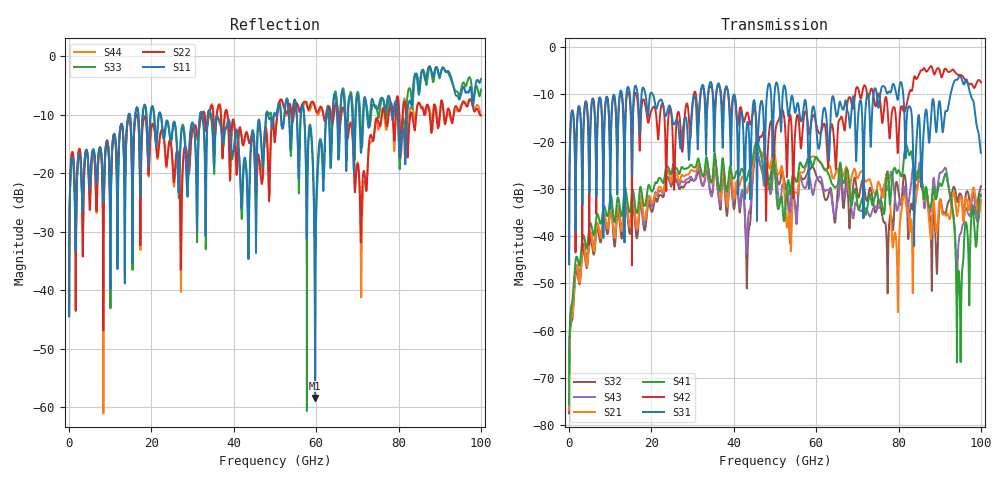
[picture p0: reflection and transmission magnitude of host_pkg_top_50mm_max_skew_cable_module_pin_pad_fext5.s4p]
# Hz S RI R 50
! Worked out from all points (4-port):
!   10000 points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, 10 MHz to 100 GHz, reference 50 ohm
!   strongest paths, dB at 10 MHz, 25.01 GHz, 50.01 GHz, 75.01 GHz, 100 GHz:
!     S31: -46.0, -15.0, -8.7, -12.4, -22.4
!     S42: -45.9, -16.0, -18.9, -10.1, -7.5
!     S41: -75.7, -26.1, -26.6, -32.0, -31.5
!     S21: -76.7, -27.8, -23.0, -28.6, -32.6
!     S43: -76.8, -28.1, -25.4, -34.0, -32.4
!     S32: -77.5, -28.8, -24.1, -32.7, -29.5
!   lowest |S11| = -58.4 dB at 59.73 GHz (marker M1), VSWR 1.00, Z = 50.1 + j0.0909 ohm
!   |S11| at or under -10 dB: start of sweep to 14.44 GHz; 22.24 GHz to 31.79 GHz (9.548 GHz wide, 35.3 % of centre); 34.36 GHz to 47.86 GHz (13.5 GHz wide, 32.8 % of centre)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
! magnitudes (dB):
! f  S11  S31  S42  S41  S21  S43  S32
! 10 MHz  -44.4  -46.0  -45.9  -75.7  -76.7  -76.8  -77.5
! 10.07 GHz  -31.9  -26.7  -21.5  -31.6  -33.2  -33.0  -33.9
! 52.9 GHz  -7.3  -11.9  -27.5  -29.9  -38.2  -29.5  -30.6
! 59.73 GHz  -58.4  -14.2  -15.1  -23.6  -23.2  -29.1  -26.4
! 91.47 GHz  -2.6  -13.5  -4.6  -26.8  -35.7  -25.7  -35.1
! 94.65 GHz  -7.3  -6.3  -5.9  -47.6  -33.1  -40.9  -31.5
! 100 GHz  -3.9  -22.4  -7.5  -31.5  -32.6  -32.4  -29.5
